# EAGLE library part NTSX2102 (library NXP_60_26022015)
Dual supply translating transceiver; open drain; auto direction sensing The NTSX2102 is a 2-bit, dual supply translating transceiver with auto direction sensing, that enables bidirectional voltage level translation. It features two 2-bit input-output ports (An and Bn), one output enable input (OE) and two supply pins (VCC(A) and VCC(B)). Both supplies can be supplied at any voltage between 1.65 V and 5.5 V. This flexibility makes the device suitable for translating between any of the voltage nodes (1.8 V, 2.5 V, 3.3 V and 5.0 V). Pins An and OE are referenced to VCC(A) and pins Bn are referenced to VCC(B). A LOW level at pin OE causes the outputs to assume a high-impedance OFF-state. This device is fully specified for partial power-down applications using IOFF. The IOFF circuitry disables the output, preventing the damaging backflow current through the device when it is powered down. AAL Eindhoven MK
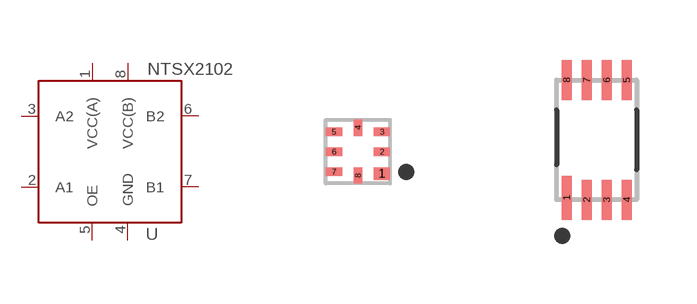
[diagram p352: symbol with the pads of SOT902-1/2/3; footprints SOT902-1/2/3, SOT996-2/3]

Designator prefix -

## NTSX2102GM  [SOT902-1/2/3]
1  VCC(A)  out
2  A1  out
3  A2  out
4  GND  out
5  OE  out
6  B2  out
7  B1  out
8  VCC(B)  out

## NTSX2102GD  [SOT996-2/3]
Pads as for SOT902-1/2/3

## Footprint SOT902-1/2/3 (pad centres in mm)
SOT902-1/2/3 XQFN8U: plastic extremely thin quad flat package; no leads; 8 terminals; UTLP based; body 1.6 x 1.6 x 0.5 mm JEDEC: -- IEC: ---
smd 0.4 x 0.32: 1 0.6,-0.55
smd 0.4 x 0.22: 2 0.6,0; 3 0.6,0.5; 5 -0.6,0.5; 6 -0.6,0; 7 -0.6,-0.5
smd 0.22 x 0.4: 4 0,0.6; 8 0,-0.6

## Footprint SOT996-2/3 (pad centres in mm)
SOT996-2/3 XSON8U: plastic extremely thin small outline package; no leads;8 terminals; UTLP based; body 3 x 2 x 0.5 mm JEDEC: IEC: -- JEITA: --
smd 0.25 x 1.1: 1 -0.75,-1.45
smd 0.25 x 1: 2 -0.25,-1.5; 3 0.25,-1.5; 4 0.75,-1.5; 5 0.75,1.5; 6 0.25,1.5; 7 -0.25,1.5; 8 -0.75,1.5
